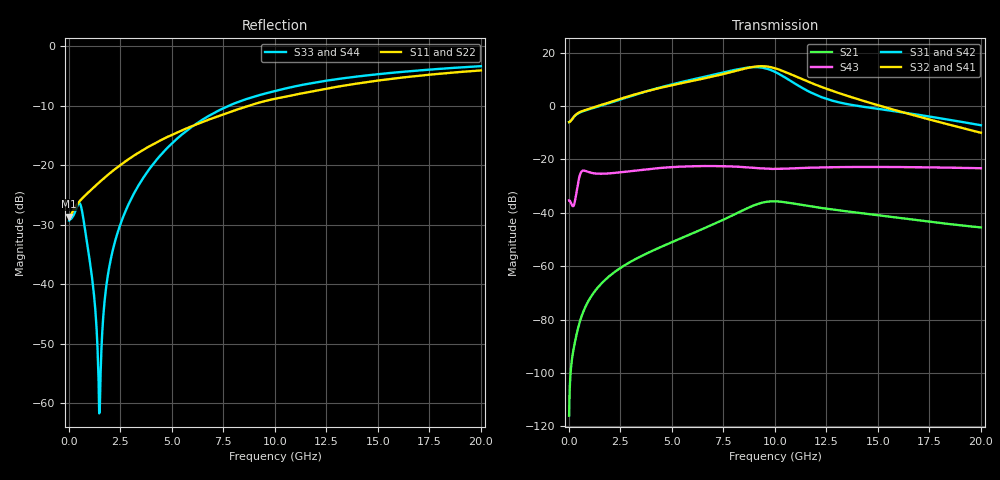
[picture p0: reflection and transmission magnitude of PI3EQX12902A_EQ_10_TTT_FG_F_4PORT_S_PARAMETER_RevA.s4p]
! NPort=4 DATA=2000 NOISE=0 GROUPDELAY=0 COMPLEX_DATAFORMAT=POLAR
! NumOfBlock=1 NumOfParam=0
! .MODEL Smodel S TSTONEFILE=PI3EQX12902A_EQ_10_TTT_FG_F_4PORT_S_PARAMETER_RevA.s4p TYPE=S
!  -- The above .MODEL line can be used for the S element in the netlist.
! The s parameter is extracted from the linear redriver, it is not bi-directional; only s(4,1)s(4,2) and s(3,1)s(3,2)
! should be the insertion loss
!Port definition:
!Port1 = input+
!Port2 = input-
!Port3 = output+
!Port4 = output-
# Hz S MA R  50
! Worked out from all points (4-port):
!   2000 points, 10 MHz to 20 GHz, reference 50 ohm
!   strongest paths, dB at 10 MHz, 5.01 GHz, 10.01 GHz, 15.01 GHz, 20 GHz:
!     S32: -6.0, 7.8, 14.1, 0.3, -10.0
!     S41: -6.0, 7.8, 14.1, 0.3, -10.0
!     S31: -6.0, 8.1, 12.8, -1.1, -7.2
!     S42: -6.0, 8.0, 12.6, -1.3, -7.4
!     S43: -35.3, -22.9, -23.6, -22.8, -23.3
!     S21: -116.0, -51.0, -35.7, -40.9, -45.5
!   lowest |S11| = -28.6 dB at 10 MHz (marker M1), VSWR 1.08, Z = 46.4 - j0.0607 ohm
!   |S11| at or under -10 dB: start of sweep to 8.737 GHz
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1e7  0.03704 -179.0  1.589e-06 51.9  0 0.0  0 0.0
     1.589e-06 51.9  0.03704 -179.0  0 0.0  0 0.0
     0.4991 1.1  0.4991 -178.9  0.03429 6.0  0.01709 -177.1
     0.4991 -178.9  0.4991 1.1  0.01709 -177.1  0.03429 6.0
5.98e9  0.2129 -111.8  0.004094 98.9  1.631e-06 -22.1  9.887e-07 86.6
        0.004093 98.8  0.2129 -111.8  9.913e-07 86.8  1.625e-06 -21.8
        3.131 -52.2  2.945 108.8  0.2108 -46.2  0.07402 144.9
        2.935 108.7  3.092 -52.7  0.07442 145.0  0.2102 -46.3
8.14e9  0.2925 -111.7  0.009759 76.6  8.14e-06 -85.5  4.908e-06 42.0
        0.009755 76.6  0.2925 -111.7  4.933e-06 42.1  8.12e-06 -85.1
        4.82 -111.3  4.588 50.5  0.3363 -67.4  0.07258 122.2
        4.565 50.4  4.75 -111.6  0.07305 122.1  0.3356 -67.3
9.34e9  0.3399 -113.6  0.0153 45.3  1.457e-05 -133.2  1.172e-05 -2.9
        0.01532 45.3  0.3399 -113.6  1.178e-05 -2.9  1.457e-05 -132.7
        5.257 -162.8  5.567 -0.1  0.392 -76.9  0.06741 113.2
        5.53 -0.1  5.186 -163.1  0.0678 113.0  0.3916 -76.8
1.045e10  0.3745 -115.8  0.01583 9.2  1.567e-05 -172.1  1.691e-05 -55.7
          0.01586 9.2  0.3745 -115.8  1.698e-05 -55.7  1.571e-05 -171.6
          3.502 148.9  4.422 -52.2  0.4387 -84.0  0.06665 109.3
          4.39 -52.0  3.456 148.4  0.06691 109.0  0.4386 -83.9
1.245e10  0.4372 -118.6  0.01201 -25.7  1.868e-05 160.4  1.917e-05 -121.2
          0.01204 -25.9  0.4372 -118.6  1.921e-05 -121.2  1.876e-05 160.7
          1.38 118.0  2.138 -108.8  0.5117 -95.0  0.07094 96.5
          2.128 -108.4  1.349 117.4  0.07096 96.2  0.512 -94.9
2e10  0.6257 -131.7  0.005357 -76.2  3.997e-05 51.2  1.805e-05 96.3
      0.005324 -76.5  0.6257 -131.7  1.804e-05 96.4  4.012e-05 51.3
      0.4364 36.8  0.3155 129.4  0.6794 -119.6  0.06842 46.2
      0.3176 129.7  0.4281 37.4  0.06833 46.1  0.6797 -119.6
